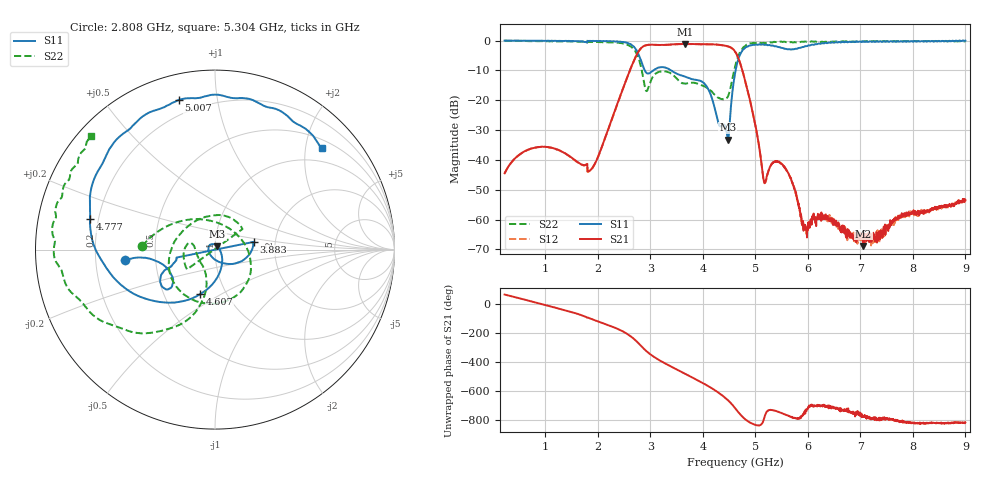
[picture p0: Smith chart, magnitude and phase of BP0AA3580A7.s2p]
!Agilent Technologies,E8358A,US41080443,A.07.50.56
!Agilent E8358A: A.07.50.56
!Date: Wednesday, May 23, 2018 14:55:51
!Correction: S11(Full 2 Port(1,2))
!S21(Full 2 Port(1,2))
!S12(Full 2 Port(1,2))
!S22(Full 2 Port(1,2))
!S2P File: Measurements: S11, S21, S12, S22:
# Hz S  dB  R 50
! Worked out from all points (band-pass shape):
!   1601 points, 225 MHz to 9 GHz, reference 50 ohm
!   highest |S21| = -1.14 dB at 3.669 GHz (marker M1); lowest = -68.8 dB at 7.059 GHz (marker M2)
!   |S21| within 3 dB of the highest: 2.758 GHz to 4.631 GHz (1.872 GHz wide, 50.7 % of centre)
!   lowest |S11| = -33.2 dB at 4.475 GHz (marker M3), VSWR 1.04, Z = 51.2 + j1.84 ohm
!   |S11| at or under -10 dB: 2.894 GHz to 3.059 GHz (164.8 MHz wide, 5.53 % of centre); 3.393 GHz to 4.623 GHz (1.23 GHz wide, 30.7 % of centre)
!   |S22| runs from -19.8 to -0.1 dB; largest |S21 - S12| = 0.0072
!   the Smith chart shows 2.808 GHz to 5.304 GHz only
!   S11 on the Smith chart (normalised r, x): 2.808 GHz: 0.33, -0.05; 3.883 GHz: 1.54, +0.14; 4.607 GHz: 0.75, -0.40; 4.777 GHz: 0.17, +0.12; 5.007 GHz: 0.12, +0.78; 5.304 GHz: 0.67, +2.33
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2.25e8  -0.02 -8.3  -44.47 67.3  -44.52 67.5  -0.08 -34.3
6.308438e8  -0.07 -23.9  -36.92 29.7  -36.96 29.9  -0.17 -95.3
1.069594e9  -0.08 -43.5  -35.72 -11.9  -35.83 -11.8  -0.28 -160.5
1.689328e9  -0.33 -85.9  -41.56 -74.8  -41.53 -75.3  -0.32 113.5
2.215828e9  -0.24 -98.4  -28.86 -145.8  -28.89 -146.2  -0.65 -1.1
2.566828e9  -0.81 -135.3  -12.00 154.3  -12.03 154.7  -1.43 -80.0
2.808141e9  -5.97 -173.2  -2.83 79.2  -2.90 79.2  -7.84 177.3
3.153656e9  -9.05 -141.2  -1.44 -21.3  -1.51 -21.2  -10.56 -81.3
3.669188e9  -12.15 -161.1  -1.14 -119.9  -1.21 -119.9  -14.48 102.4
3.883078e9  -13.20 11.3  -1.18 -160.1  -1.24 -160.0  -14.38 -144.7
4.475391e9  -33.17 54.7  -1.93 60.4  -1.96 60.4  -18.87 -126.4
4.607016e9  -11.65 -108.5  -3.54 8.1  -3.58 8.1  -9.30 -106.2
4.6125e9  -11.06 -111.6  -3.67 5.8  -3.71 5.8  -8.87 -107.0
4.777031e9  -2.89 166.3  -11.56 -63.1  -11.56 -63.0  -2.17 -153.4
5.007375e9  -1.33 103.7  -28.94 -110.9  -29.05 -111.0  -0.82 167.3
5.166422e9  -1.44 71.6  -47.34 -67.1  -47.31 -67.8  -0.81 149.9
5.303531e9  -1.72 43.6  -41.48 -8.1  -41.49 -7.8  -0.59 137.5
5.714859e9  -2.92 -83.9  -48.15 -60.5  -48.36 -60.1  -0.65 111.6
6.076828e9  -1.38 -179.2  -59.56 28.6  -60.08 25.9  -0.27 89.5
7.058531e9  -0.30 101.3  -68.84 -51.7  -65.88 -49.5  -0.29 40.2
7.541156e9  -0.41 82.1  -62.27 -66.5  -62.37 -65.6  -0.31 20.2
9e9  -0.06 48.8  -53.44 -94.2  -53.49 -94.7  -0.30 -21.4
